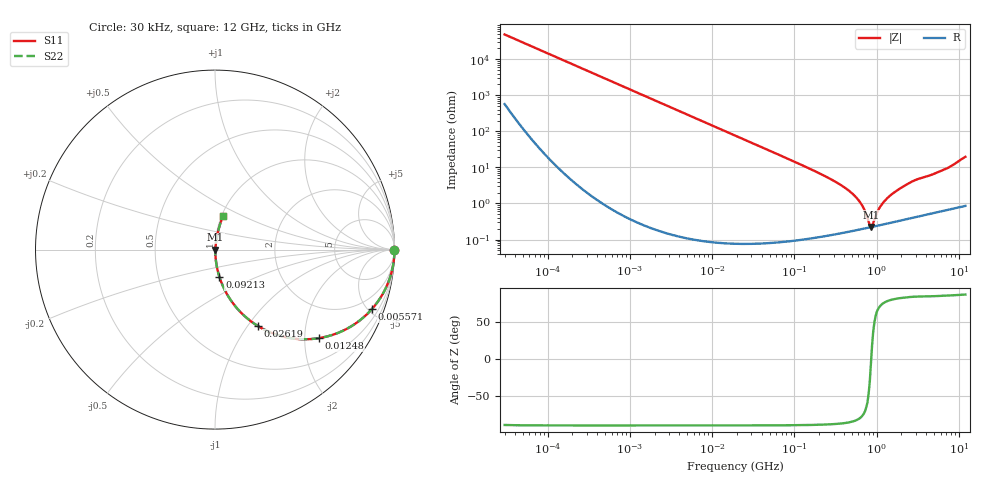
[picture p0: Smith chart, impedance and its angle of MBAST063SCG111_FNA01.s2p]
! MBAST063SCG111_FNA01  S-PARAMETER MODEL  ( General Type )
! Model Generated by TAIYO YUDEN Corporation (http://www.ty-top.com)
! Version 1.0
! TAIYO YUDEN Control No. 130801
! Copyright(c) 2013 TAIYO YUDEN CO.,LTD. All Rights Reserved.
! Product Description (link to TY-COMPAS)
! https://ds.yuden.co.jp/TYCOMPAS/or/detail?pn=MBAST063SCG111JFNA01&u=M
! Products Name : Multilayer Ceramic Capacitors
! Characteristics :
!  Capacitance : 110 pF , Rated Voltage : 25V , TCC : CG / C0G
!  Case Size : 0.6 x 0.3 / 0.024 x 0.012 [mm/inch] , Thickness : 0.3 / 0.012 [mm/inch]
!  (Conditions: Temperature = 25 degC , DC Bias Current/Voltage = 0A / 0V)
! External Node Assignments :
!  1  o---| |---o  2
! GND o---------o GND
! Frequency Range : 0.03MHz  -  12000MHz  [ 401 STEP ]
# MHz S RI R 50
! Freq[MHz].  S11 Real  S11 Imag  S21 Real  S21 Imag  S12 Real  S12 Imag  S22 Real  S22 Imag
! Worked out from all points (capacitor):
!   401 points, 30 kHz to 12 GHz, reference 50 ohm
!   read as one part in series: C = 109 pF near 32 kHz
!   lowest |Z| = 222 mohm at 852.6 MHz (marker M1)
!   series resonance near 860.1 MHz, so ESL is about 310 pH
!   S11 on the Smith chart (normalised r, x): 30 kHz: open; 5.571 MHz: 1.00, -5.25; 12.48 MHz: 1.00, -2.34; 26.19 MHz: 1.00, -1.12; 92.13 MHz: 1.00, -0.31; 12 GHz: 1.02, +0.39
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0.03  1 -0.00205  2.83e-05 0.00205  2.83e-05 0.00205  1 -0.00205
0.260295  0.9997 -0.0178  0.000325 0.0178  0.000325 0.0178  0.9997 -0.0178
0.915519  0.9961 -0.0624  0.00392 0.0624  0.00392 0.0624  0.9961 -0.0624
2.258455  0.9766 -0.1509  0.0234 0.1509  0.0234 0.1509  0.9766 -0.1509
5.571287  0.8731 -0.3327  0.1269 0.3327  0.1269 0.3327  0.8731 -0.3327
12.47626  0.5784 -0.4935  0.4216 0.4935  0.4216 0.4935  0.5784 -0.4935
18.97367  0.3724 -0.4829  0.6276 0.4829  0.6276 0.4829  0.3724 -0.4829
26.19406  0.2374 -0.4248  0.7626 0.4248  0.7626 0.4248  0.2374 -0.4248
45.32004  0.0943 -0.2911  0.9057 0.2911  0.9057 0.2911  0.0943 -0.2911
92.13054  0.0248 -0.1528  0.9752 0.1528  0.9752 0.1528  0.0248 -0.1528
164.6252  0.00832 -0.0847  0.9917 0.0847  0.9917 0.0847  0.00832 -0.0847
334.6645  0.00279 -0.0368  0.9972 0.0368  0.9972 0.0368  0.00279 -0.0368
508.9517  0.00206 -0.0185  0.9979 0.0185  0.9979 0.0185  0.00206 -0.0185
658.7456  0.00202 -0.00898  0.998 0.00898  0.998 0.00898  0.00202 -0.00898
799.3715  0.00213 -0.00228  0.9979 0.00228  0.9979 0.00228  0.00213 -0.00228
852.6267  0.0022 -0.000272  0.9978 0.000272  0.9978 0.000272  0.0022 -0.000272
909.4299  0.00227 0.00174  0.9977 -0.00174  0.9977 -0.00174  0.00227 0.00174
1103.571  0.00256 0.00766  0.9974 -0.00766  0.9974 -0.00766  0.00256 0.00766
1428.372  0.00309 0.0155  0.9969 -0.0155  0.9969 -0.0155  0.00309 0.0155
2635.962  0.00543 0.039  0.9946 -0.039  0.9946 -0.039  0.00543 0.039
6715.658  0.0138 0.0859  0.9862 -0.0859  0.9862 -0.0859  0.0138 0.0859
12000  0.045 0.1867  0.955 -0.1867  0.955 -0.1867  0.045 0.1867
